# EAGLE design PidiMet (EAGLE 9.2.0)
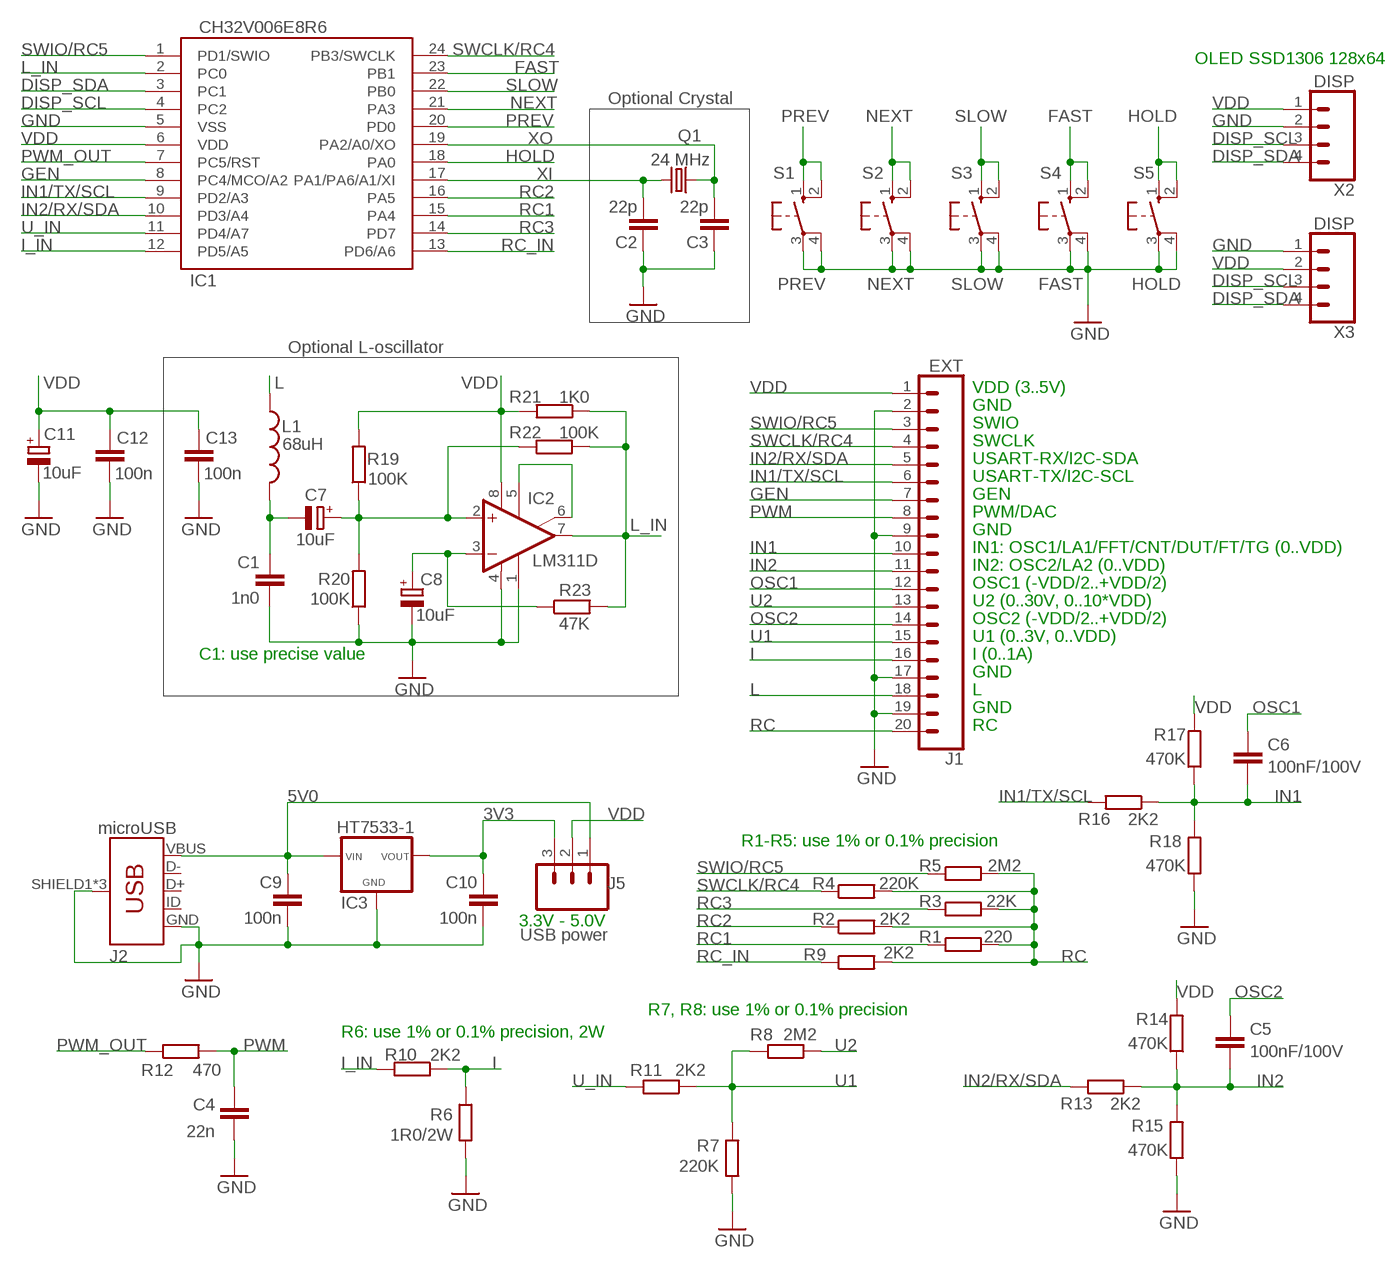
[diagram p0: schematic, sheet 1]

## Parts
C1  1n0  C5/2.5  [C5B2.5]
C2  22p  C-EUC1206  [C1206]
C3  22p  C-EUC1206  [C1206]
C4  22n  C-EUC1206  [C1206]
C5  100nF/100V  C-EUC1206  [C1206]
C6  100nF/100V  C-EUC1206  [C1206]
C7  10uF  CPOL-EUTT2D4L  [TT2D4L]
C8  10uF  CPOL-EUTT2D4L  [TT2D4L]
C9  100n  C-EUC1206  [C1206]
C10  100n  C-EUC1206  [C1206]
C11  10uF  CPOL-EUTT2D4L  [TT2D4L]
C12  100n  C-EUC1206  [C1206]
C13  100n  C-EUC1206  [C1206]
IC1  CH32V006E8R6  CH32V006E8R6CH32V006E8R6_2  [QSOP24_2]
IC2  LM311D  [SO08]
IC3  HT7533-1  [HT7533-1]
J1  EXT  CONN_201X20_LONGPADS  [1X20_LONGPADS]
J2  microUSB  USB_MICRO-B  [USB-B-MICRO-SMD_2]
J5  USB power  CONN_03LONGPADS  [1X03_LONGPADS]
L1  68uH  L-USLAL04  [LAL04]
Q1  24 MHz  CRYSTALHC49U-V  [HC49U-V]
R1  220  R-EU_0204/5  [0204/5]
R2  2K2  R-EU_0204/5  [0204/5]
R3  22K  R-EU_0204/5  [0204/5]
R4  220K  R-EU_0204/5  [0204/5]
R5  2M2  R-EU_0204/5  [0204/5]
R6  1R0/2W  R-EU_0414/15  [0414/15]
R7  220K  R-EU_0204/7  [0204/7]
R8  2M2  R-EU_0204/7  [0204/7]
R9  2K2  R-EU_R1206  [R1206]
R10  2K2  R-EU_R1206  [R1206]
R11  2K2  R-EU_R1206  [R1206]
R12  470  R-EU_R1206  [R1206]
R13  2K2  R-EU_R1206  [R1206]
R14  470K  R-EU_R1206  [R1206]
R15  470K  R-EU_R1206  [R1206]
R16  2K2  R-EU_R1206  [R1206]
R17  470K  R-EU_R1206  [R1206]
R18  470K  R-EU_R1206  [R1206]
R19  100K  R-EU_R1206  [R1206]
R20  100K  R-EU_R1206  [R1206]
R21  1K0  R-EU_R1206  [R1206]
R22  100K  R-EU_R1206  [R1206]
R23  47K  R-EU_R1206  [R1206]
S1  PREV  10-XX  [B3F-10XX]
S2  NEXT  10-XX  [B3F-10XX]
S3  SLOW  10-XX  [B3F-10XX]
S4  FAST  10-XX  [B3F-10XX]
S5  HOLD  10-XX  [B3F-10XX]
X2  DISP  CONN_04  [1X04]
X3  DISP  CONN_04  [1X04]

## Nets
3V3: C10.2 IC3.VOUT J5.3
5V0: C9.2 IC3.VIN J2.VBUS J5.1
DISP_SCL: IC1.4(PC2) X2.3 X3.3
DISP_SDA: IC1.3(PC1) X2.4 X3.4
FAST: IC1.23(PB1) S4.1(S) S4.2(S1)
GEN: IC1.8(PC4/MCO/A2) J1.7
GND: C1.2 C2.1 C3.1 C4.1 C8.- C9.1 C10.1 C11.- C12.1 C13.1 IC1.5(VSS) IC2.1(GND) IC2.4(V-) IC3.GND J1.2 J1.9 J1.17 J1.19 J2.GND J2.SHIELD1(SHIELD) J2.SHIELD2(SHIELD) J2.SHIELD3(SHIELD) R6.2 R7.2 R15.1 R18.1 R20.1 S1.3(P) S1.4(P1) S2.3(P) S2.4(P1) S3.3(P) S3.4(P1) S4.3(P) S4.4(P1) S5.3(P) S5.4(P1) X2.2 X3.1
HOLD: IC1.18(PA0) S5.1(S) S5.2(S1)
I: J1.16 R6.1 R10.1
I_IN: IC1.12(PD5/A5) R10.2
IN1: C6.2 J1.10 R16.1 R17.1 R18.2
IN1/TX/SCL: IC1.9(PD2/A3) J1.6 R16.2
IN2: C5.2 J1.11 R13.1 R14.1 R15.2
IN2/RX/SDA: IC1.10(PD3/A4) J1.5 R13.2
L: J1.18 L1.1
L_IN: IC1.2(PC0) IC2.7(OUT) R21.1 R22.2 R23.2
N$8: C7.+ IC2.2(+IN) R19.1 R20.2 R22.1
N$9: C1.1 C7.- L1.2
N$11: C8.+ IC2.3(-IN) R23.1
N$15: IC2.5(ON) IC2.6(ON/STR)
NEXT: IC1.21(PA3) S2.1(S) S2.2(S1)
OSC1: C6.1 J1.12
OSC2: C5.1 J1.14
PREV: IC1.20(PD0) S1.1(S) S1.2(S1)
PWM: C4.2 J1.8 R12.2
PWM_OUT: IC1.7(PC5/RST) R12.1
RC: J1.20 R1.2 R2.2 R3.2 R4.2 R5.2 R9.2
RC1: IC1.15(PA4) R1.1
RC2: IC1.16(PA5) R2.1
RC3: IC1.14(PD7) R3.1
RC_IN: IC1.13(PD6/A6) R9.1
SLOW: IC1.22(PB0) S3.1(S) S3.2(S1)
SWCLK/RC4: IC1.24(PB3/SWCLK) J1.4 R4.1
SWIO/RC5: IC1.1(PD1/SWIO) J1.3 R5.1
U1: J1.15 R7.1 R8.2 R11.1
U2: J1.13 R8.1
U_IN: IC1.11(PD4/A7) R11.2
VDD: C11.+ C12.2 C13.2 IC1.6(VDD) IC2.8(V+) J1.1 J5.2 R14.2 R17.2 R19.2 R21.2 X2.1 X3.2
XI: C2.2 IC1.17(PA1/PA6/A1/XI) Q1.2
XO: C3.2 IC1.19(PA2/A0/XO) Q1.1
Unconnected: J2.D+ J2.D- J2.ID

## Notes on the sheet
- OLED SSD1306 128x64
- Optional Crystal
- Optional L-oscillator
- VDD (3..5V)
- GND
- SWIO
- SWCLK
- USART-RX/I2C-SDA
- USART-TX/I2C-SCL
- GEN
- PWM/DAC
- GND
- IN1: OSC1/LA1/FFT/CNT/DUT/FT/TG (0..VDD)
- IN2: OSC2/LA2 (0..VDD)
- OSC1 (-VDD/2..+VDD/2)
- U2 (0..30V, 0..10*VDD)
- OSC2 (-VDD/2..+VDD/2)
- U1 (0..3V, 0..VDD)
- C1: use precise value | I (0..1A)
- GND
- L
- GND
- RC
- R1-R5: use 1% or 0.1% precision
- 3.3V - 5.0V
- R7, R8: use 1% or 0.1% precision
- R6: use 1% or 0.1% precision, 2W

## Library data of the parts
C1 = capacitor-wima:C: CAPACITOR
C2-C6 C9 C10 C12 C13 = rcl:C-EU: CAPACITOR, European symbol; SPICEPREFIX: C
C7 C8 C11 = rcl:CPOL-EU: POLARIZED CAPACITOR, European symbol; SPICEPREFIX: C
IC1 = CH32V:CH32V006E8R6
IC2 = linear:LM311: COMPARATOR
IC3 = HT7533-1B:HT7533-1
J1 = SparkFun-Connectors:CONN_20: Multi connection point. Often used as Generic Header-pin footprint for 0.1 inch spaced/style header connections On any of the 0.1 inch spaced packages, you can populate with these: Break Away Headers - Straight (PRT-00116) Break Away Male Headers - Right Angle (PRT-00553) Female Headers (PRT-00115)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
J2 = SparkFun-Connectors:USB_MICRO-B: USB Type Micro-B Connector Male/female and PTH/SMT variants SparkFun Products: SparkFun microB USB Breakout SparkFun USB microB Plug Breakout SparkFun ESP8266 Thing
J5 = SparkFun-Connectors:CONN_03: Multi connection point. Often used as Generic Header-pin footprint for 0.1 inch spaced/style header connections On any of the 0.1 inch spaced packages, you can populate with these: Break Away Headers - Straight (PRT-00116) Break Away Male Headers - Right Angle (PRT-00553) Female Headers (PRT-00115)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
L1 = rcl:L-US: INDUCTOR, American symbol; SPICEPREFIX: L
Q1 = crystal:CRYSTAL: CRYSTAL; OC_FARNELL: 1666969; OC_NEWARK: unknown
R1-R23 = rcl:R-EU_: RESISTOR, European symbol; SPICEPREFIX: R
S1-S5 = switch-omron:10-XX: OMRON SWITCH; MPN: B3F-1000; OC_FARNELL: 176432; OC_NEWARK: 36M3542
X2 X3 = SparkFun-Connectors:CONN_04: Multi connection point. Often used as Generic Header-pin footprint for 0.1 inch spaced/style header connections On any of the 0.1 inch spaced packages, you can populate with these: Break Away Headers - Straight (PRT-00116) Break Away Male Headers - Right Angle (PRT-00553) Female Headers (PRT-00115)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; PROD_ID: CONN-09696

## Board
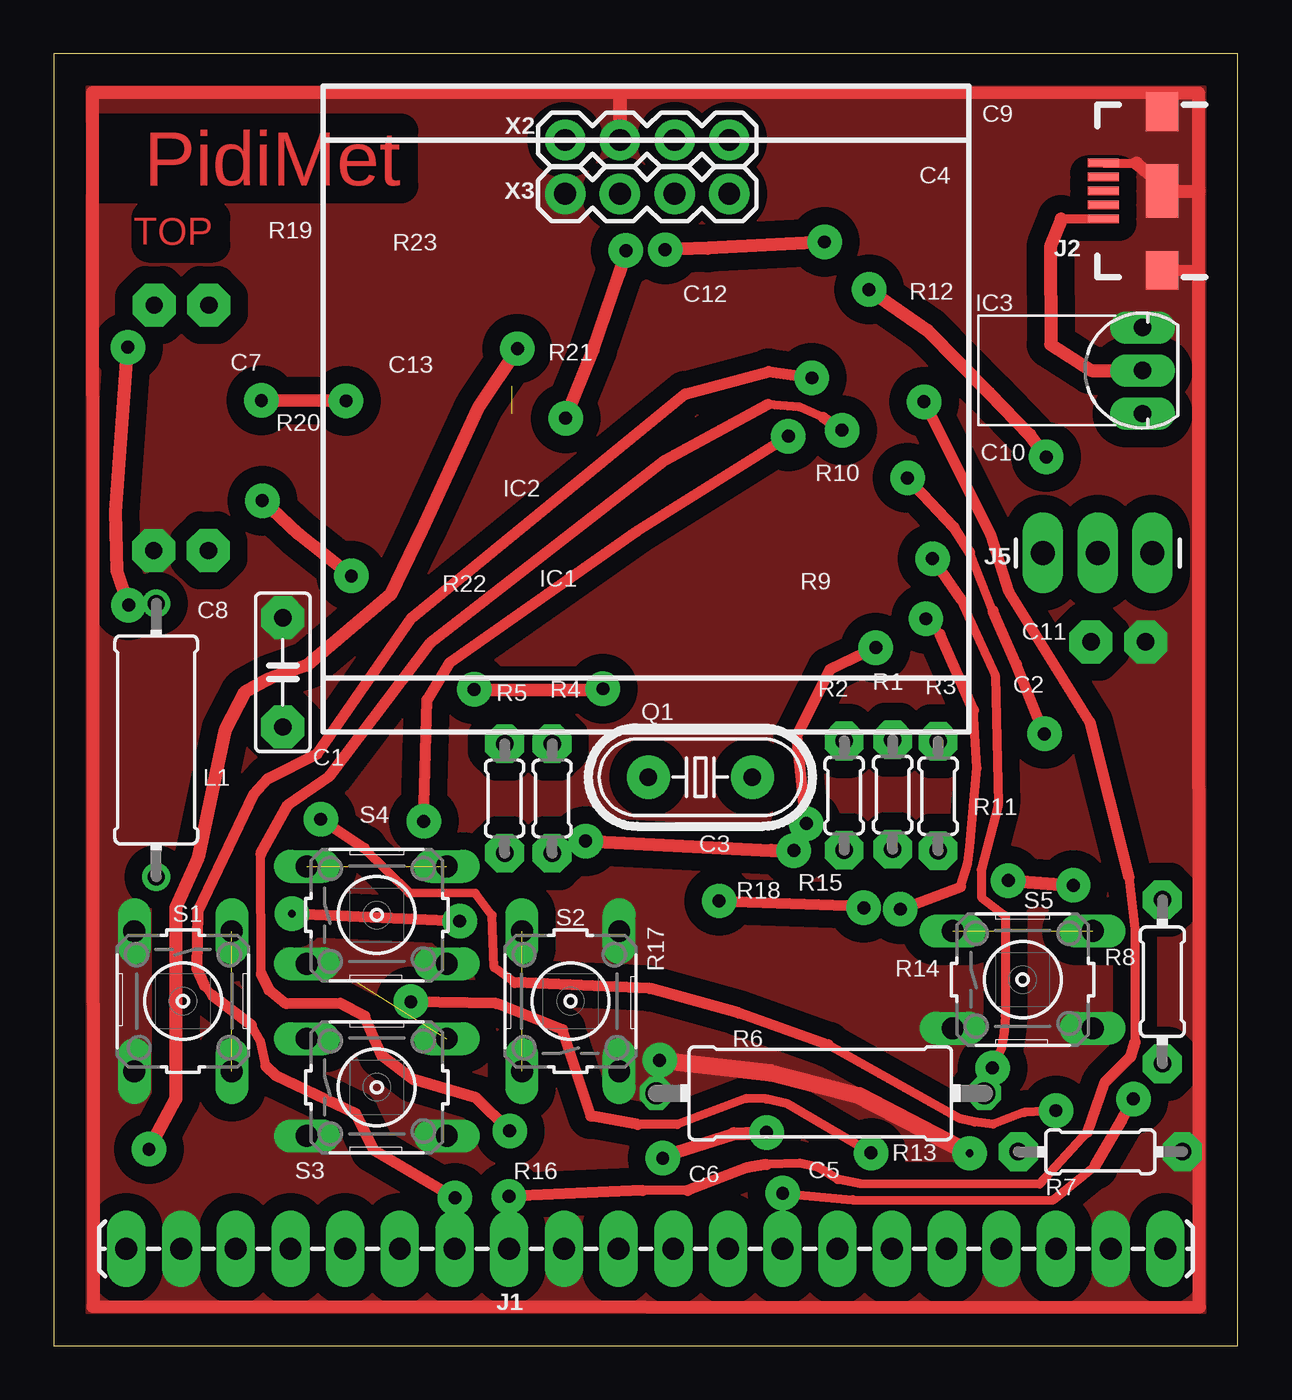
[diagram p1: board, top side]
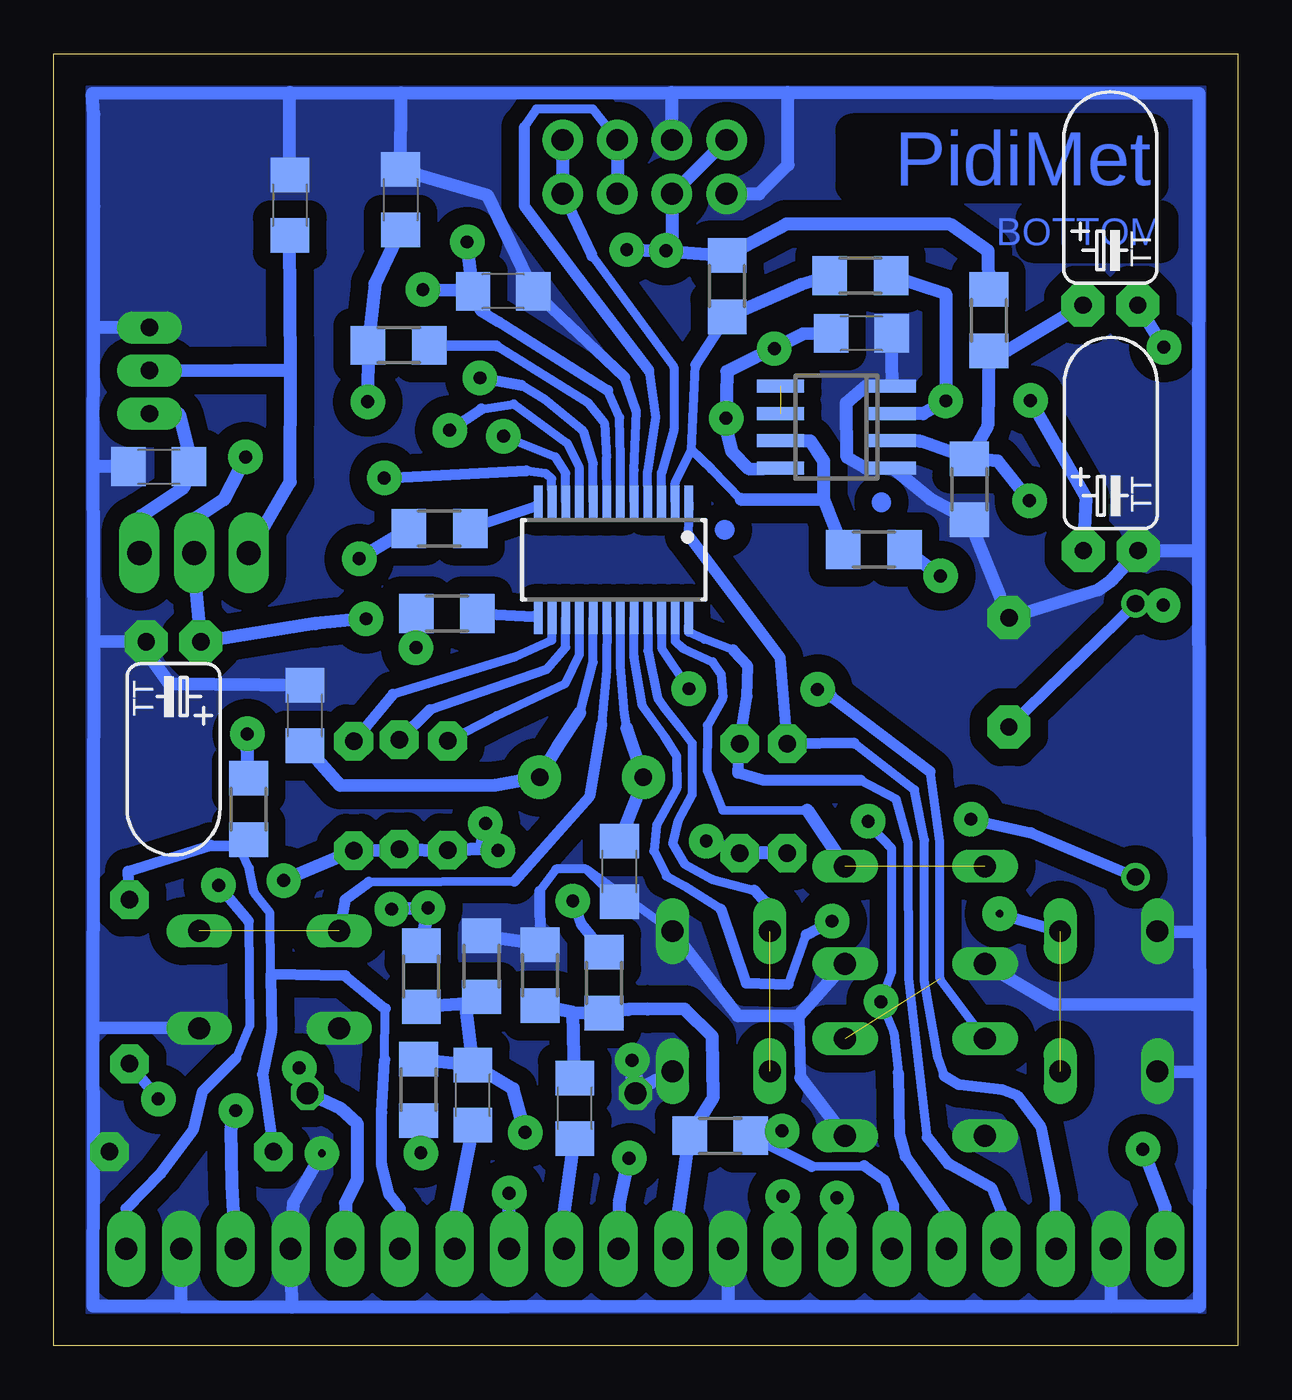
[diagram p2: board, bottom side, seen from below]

Size 55 x 60 mm. Coordinates in mm from the lower left corner, seen from the top.
Outline: 0,0 55,0 55,60 0,60 0,0
Copper layers (1*16): Top 0.035mm / dielectric 1.5mm / Bottom 0.035mm
Design rules "default": minimum track width 6mil, minimum drill 0.35mm, track to track 6mil, track to pad 6mil, pad to pad 6mil, via to via 6mil, smd to smd 6mil, copper to edge 40mil, drill to drill 6mil, minimum pad ring 10mil, minimum via ring 8mil, stop-mask expansion 4mil, vias tented up to drill 0mil, thermal gap 10mil

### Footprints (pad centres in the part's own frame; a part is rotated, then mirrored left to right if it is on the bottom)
C5B2.5 = drill 0.8 pad 2 octagon: 1 -2.54,0 | drill 0.813 pad 2 octagon: 2 2.54,0
C1206 = smd 1.6 x 1.8: 1 -1.4,0; 2 1.4,0
TT2D4L = drill 0.8 pad 2 octagon: + -1.27,0; - 1.27,0
QSOP24_2 = smd 0.4 x 1.5: 1 -3.493,-2.69; 2 -2.857,-2.69; 3 -2.223,-2.69; 4 -1.587,-2.69; 5 -0.953,-2.69; 6 -0.318,-2.69; 7 0.318,-2.69; 8 0.953,-2.69; 9 1.587,-2.69; 10 2.223,-2.69; 11 2.857,-2.69; 12 3.493,-2.69; 13 3.493,2.69; 14 2.857,2.69; 15 2.223,2.69; 16 1.587,2.69; 17 0.953,2.69; 18 0.318,2.69; 19 -0.318,2.69; 20 -0.953,2.69; 21 -1.587,2.69; 22 -2.223,2.69; 23 -2.857,2.69; 24 -3.493,2.69
SO08 = smd 0.6 x 2.2: 1 -1.905,-2.6; 2 -0.635,-2.6; 3 0.635,-2.6; 4 1.905,-2.6; 5 1.905,2.6; 6 0.635,2.6; 7 -0.635,2.6; 8 -1.905,2.6
HT7533-1 = drill 0.8 pad 1.5 long: GND 2,0; VIN 0,0; VOUT -2,0
1X20_LONGPADS = drill 1.016 pad 1.778 long: 1 -24.13,0; 2 -21.59,0; 3 -19.05,0; 4 -16.51,0; 5 -13.97,0; 6 -11.43,0; 7 -8.89,0; 8 -6.35,0; 9 -3.81,0; 10 -1.27,0; 11 1.27,0; 12 3.81,0; 13 6.35,0; 14 8.89,0; 15 11.43,0; 16 13.97,0; 17 16.51,0; 18 19.05,0; 19 21.59,0; 20 24.13,0
USB-B-MICRO-SMD_2 = smd 1.45 x 0.4: D+ 2.725,0; D- 2.725,0.65; GND 2.725,-1.3; ID 2.725,-0.65; VBUS 2.725,1.3 | smd 1.5 x 1.8: SHIELD1 0,3.685; SHIELD2 0,-3.685 | smd 1.5 x 2.5: SHIELD3 0,0
1X03_LONGPADS = drill 1.118 pad 1.88 long: 1 0,0; 2 2.54,0; 3 5.08,0
LAL04 = drill 0.8 pad 1.3: 1 -6.35,0; 2 6.35,0
HC49U-V = drill 0.813 pad 2: 1 -2.413,0; 2 2.413,0
0204/5 = drill 0.813 pad 1.8 octagon: 1 -2.54,0; 2 2.54,0
0414/15 = drill 1.016 octagon: 1 -7.62,0; 2 7.62,0
0204/7 = drill 0.813 pad 1.8 octagon: 1 -3.81,0; 2 3.81,0
R1206 = smd 1.6 x 1.803: 1 -1.422,0; 2 1.422,0
B3F-10XX = drill 1.016 long: 1 -3.251,2.261; 2 3.251,2.261; 3 -3.251,-2.261; 4 3.251,-2.261
1X04 = drill 1.016 pad 1.88: 1 0,0; 2 2.54,0; 3 5.08,0; 4 7.62,0

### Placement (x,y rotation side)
C1  10.64,31.27 90 top
C2  43.34,29.27 270 bottom
C3  28.73,22.03 90 bottom
C4  38.89,53.23 270 bottom
C5  35.54,11.64 90 bottom
C6  30.8,11.02 90 bottom
C7  5.93,48.33 0 bottom
C8  5.91,36.93 0 bottom
C9  44.04,52.97 270 bottom
C10  50.13,40.82 0 bottom
C11  49.44,32.69 180 bottom
C12  34.13,48.97 180 bottom
C13  17.49,47.01 180 bottom
IC1  29,36.5 180 bottom
IC2  18.65,42.66 90 bottom
IC3  50.56,45.29 90 top
J1  27.5,4.5 0 top
J2  51.47,53.63 180 top
J5  45.94,36.82 0 top
L1  4.76,28.12 90 top
Q1  30.03,26.4 0 top
R1  38.96,25.6 270 top
R2  36.71,25.55 270 top
R3  41.07,25.53 270 top
R4  23.14,25.41 270 top
R5  20.94,25.42 270 top
R6  35.6,11.72 180 top
R7  48.61,9.01 0 top
R8  51.49,16.9 90 top
R9  36.75,34.01 180 bottom
R10  37.08,37.95 0 bottom
R11  45.95,24.93 90 bottom
R12  38.99,46.46 180 bottom
R13  38.06,11.88 270 bottom
R14  37.93,17.16 90 bottom
R15  35.13,17.62 270 bottom
R16  24.05,9.75 0 bottom
R17  29.44,16.86 90 bottom
R18  32.42,17.21 270 bottom
R19  11.57,47.63 90 bottom
R20  12.48,39.77 90 bottom
R21  23.72,49.21 90 bottom
R22  16.91,36.98 180 bottom
R23  17.54,49.7 180 bottom
S1  6,16 270 top
S2  24,16 90 top
S3  15,12 0 top
S4  15,20 0 top
S5  45,17 0 top
X2  23.75,56 0 top
X3  23.75,53.5 0 top

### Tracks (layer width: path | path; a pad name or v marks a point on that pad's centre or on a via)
3V3
  Bottom 0.61: J5.3 50.92,38.56 48.95,39.89 C10.2 48.78,41.68 49.19,43.27 IC3.VOUT
5V0
  Top 0.406: J2.VBUS 46.79,52.33
  Top 0.61: 46.79,52.33 46.29,51.06 46.3,46.5 48.19,45.29 IC3.VIN
  Bottom 0.61: IC3.VIN 46.59,45.3 44.01,45.3 | J5.1 44.02,40.13 44.01,45.3 | 44.01,45.3 C9.2
DISP_SCL
  Bottom 0.406: IC1.4 27.42,40.63 27.05,43.13 27.36,45.29 | X2.3 29.97,57.43 32.58,57.43 33.15,56.59
  Bottom 0.508: 33.15,56.59 33.15,52.94 30.95,50 27.36,45.29
  Bottom 0.61: X2.3 X3.3
DISP_SDA
  Bottom 0.406: IC1.3 26.78,40.53 26.2,42.54 26.2,45.45 30.01,50.62
  Bottom 0.508: X3.4 30.01,50.62
  Bottom 0.61: X2.4 X3.4
FAST  (1 unrouted)
  Bottom 0.406: IC1.23 26.14,32.72 25.77,32.38 24.4,31.76 24.01,31.19 23.93,30.09 24.65,28.81 24.65,26.7 23.93,24.87 20,24.87
  Bottom 0.61: 20,24.87 S4.2
GEN  (via drill 0.6 pad 1.6)
  Top 0.406: 9.86,12.98 9.61,14.14 9.18,14.9 | 7.36,16.27 7,16.73
  Top 0.508: v18.63,6.86 14.85,9.1 14.03,10.77 10.32,12.53 9.86,12.98 | 9.18,14.9 7.36,16.27 | 7,16.73 6.66,17.5 6.7,20.18 9.28,25.6 9.96,26.35 12.24,27.5 16.63,33.81 29.32,44.2 33.21,45.25 v35.2,44.95
  Bottom 0.406: IC1.8 29.95,40.97 30.43,42.49 32.2,43.96 33.28,44.61
  Bottom 0.508: J1.7 v18.63,6.86 | v35.2,44.95 33.28,44.61
GND  (via drill 0.35 pad 1.6, 0.6 pad 1.6)
  Top 0.406: J2.GND 50.29,54.93
  Top 0.508: J2.SHIELD2 51.45,58.17 | J2.SHIELD3 51.85,53.62 | J2.SHIELD1 53.18,49.94
  Top 0.61: 53.19,53.62 53.18,49.94 53.21,1.79 1.82,1.82 1.79,58.2 26.3,58.2 X2.2 26.29,57.99 | 53.19,53.62 53.17,58.17 51.45,58.17 26.3,58.19 26.34,58.03 | 53.19,53.62 51.85,53.62 50.29,54.93
  Top 0.813: v42.54,8.93 37.42,11.61 33.28,12.67 v28.14,13.25
  Bottom 0.406: C11.- 51.02,32.68 | IC1.5 28.04,40.67 27.94,43.39 28.48,44.98 | S2.4 30.29,22.14 | 30.29,22.14 31.68,22.14 32.43,21.11 | C3.1 30.29,22.14 | 2.1,15.85 1.78,15.81
  Bottom 0.508: 28.48,44.98 C12.1 | 32.43,21.11 R18.1 | 20.38,15.34 20.32,12.46
  Bottom 0.61: J1.19 49.11,1.83 | 49.11,1.83 43.95,1.8 | 43.95,1.8 23.7,1.86 | 23.7,1.86 5.88,1.83 | 5.88,1.83 J1.2 | J1.9 23.7,1.86 | 43.95,1.8 J1.17 43.86,6.62 v42.54,8.93 | 49.11,1.83 53.18,1.83 53.16,8.99 | 53.16,8.99 53.16,14.75 | 53.16,14.75 53.14,32.71 | 53.14,32.71 53.18,40.84 | 53.18,40.84 53.15,47.28 | 53.15,47.28 53.15,49.9 53.14,52.9 53.14,57.18 53.21,58.16 44.04,58.2 | 44.04,58.2 38.88,58.17 | 38.88,58.17 26.3,58.2 | 26.3,58.2 20.91,58.21 | 20.91,58.21 1.82,58.16 1.83,36.94 | 1.83,36.94 1.79,19.22 | 1.79,19.22 1.78,15.81 1.77,12.72 | 1.77,12.72 1.79,1.82 5.88,1.83 | S1.3 1.79,19.22 | S1.4 1.77,12.72 | S5.4 53.16,14.75 | IC3.GND 53.15,47.28 | C10.1 53.18,40.84 | 53.14,32.71 51.02,32.68 49.62,30.72 C2.1 | X2.2 26.3,58.2 | X3.1 22.24,53.5 20.89,54.85 20.91,58.21 | 27.95,11.84 S2.3 | R18.1 R15.1 | R7.2 53.16,8.99 | 1.83,36.94 C8.- 5.86,35.57 6.48,35.11 C1.2 R20.1 14.28,39.32 IC2.1 17.31,40.77 18.16,41.25 18.2,43.8 17.23,44.6 IC2.4 C13.1 | C12.1 34.86,53.43 C4.1 38.88,58.17 | S4.4 20.38,15.34 23.23,15.32 S2.4 | 20.32,12.46 S3.4 | S4.3 8.59,15.88 2.1,15.85 | C9.1 44.04,58.2
  Bottom 0.813: R6.2 27.95,11.84 v28.14,13.25
  pour Bottom (isolate 0.813, no thermals): 1.5,1.5 1.5,58.5 53.5,58.5 53.5,1.5
  pour Top (isolate 0.813, no thermals): 1.5,58.5 53.5,58.5 53.5,1.5 1.5,1.5
HOLD  (1 unrouted)
  Bottom 0.406: IC1.18 29.32,31.38 29.56,28.86 | 33.62,21.57 40.36,21.52
  Bottom 0.508: 29.56,28.86 30.13,25.5 33.62,21.57 | 40.36,21.52 41.48,20.7 S5.1
I  (via drill 0.6 pad 1.6)
  Top 0.406: 42.12,34.69 43.73,31.13 43.87,25.14 43.08,22.12 43.09,20.82 44.19,19.97 44.18,15.32 44.14,14.63 44.02,13.81 v43.6,12.89
  Top 0.508: v40.81,36.55 42.12,34.69
  Bottom 0.61: J1.16 41.45,6.63 40.9,7.74 40.89,10.29 41.65,10.99 R6.1 | R10.1 v40.81,36.55
  Bottom 0.813: R6.1 v43.6,12.89
I_IN
  Bottom 0.406: IC1.12 32.67,38.96
  Bottom 0.508: 32.67,38.96 R10.2
IN1
  Bottom 0.61: C6.2 30.87,15.47 | 30.87,15.47 R18.2 | 30.87,15.47 R17.1 28.32,15.61 27.42,15.64 25.69,15.63 24.41,14.36 24.36,11.54 R16.1 J1.10
IN1/TX/SCL  (via drill 0.6 pad 1.6)
  Top 0.406: 9.63,17.28 9.62,22.83 | 33.17,43.73 34.63,43.61 35.73,43.12
  Top 0.508: v21.17,9.97 19.6,11.52 16.69,12.37 15.22,13.48 14.45,15.3 13.3,15.9 10.79,15.88 9.99,16.51 9.63,17.28 | 9.62,22.83 10.89,25.13 12.8,26.47 17.51,32.65 28.38,41.13 33.17,43.73 | 35.73,43.12 v36.61,42.52
  Bottom 0.406: 19.79,8.33 17.36,8.36 | IC1.9 30.59,40.75 31.15,41.91 33.63,43.73 35.13,43.51 | R16.2 v21.17,9.97
  Bottom 0.508: R16.2 19.79,8.33 | 17.36,8.36 16.43,7.7 16,6.53 J1.6 | v36.61,42.52 35.13,43.51
IN2  (via drill 0.6 pad 1.6)
  Top 0.406: v28.28,8.71 28.44,8.84
  Top 0.61: 28.44,8.84 31.58,9.84 v33.11,9.9
  Bottom 0.406: 35.88,15.87 R15.2
  Bottom 0.61: C5.2 35.88,15.87 R14.1 | J1.11 28.71,6.66 v28.28,8.71 | v33.11,9.9 33.66,11.93 C5.2 | R13.1 C5.2
IN2/RX/SDA  (via drill 0.6 pad 1.6)
  Top 0.406: v37.95,8.95 34.07,11.23 33.08,11.46 32.16,11.48 28.97,10.27 27.12,10.27
  Top 0.508: 27.12,10.27 24.95,10.67 23.64,14.68 20.56,15.89 v16.58,15.97 | v17.18,24.35 17.33,29.99 18.38,31.73 27.04,37.81 v34.12,42.24
  Bottom 0.406: 15.78,12.67 15.99,14.54 v16.58,15.97 16.08,17.35 16.08,23.08 16.94,24.01 v17.18,24.35 | IC1.10 31.22,40.53 31.71,41.28 v34.12,42.24
  Bottom 0.508: R13.2 v37.95,8.95 | 15.78,12.67 15.72,9.78 15.46,8.78 13.49,6.05 J1.5
L  (via drill 0.6 pad 1.6)
  Top 0.406: v46.55,10.92 45.06,10.83 43.62,10.28 42.76,10.39 42.09,10.54 35.96,13.98 | 21.41,16.87 20.46,17.56 20.36,19.99 19.58,21.01 16.52,21.02 14.42,23.09
  Top 0.508: 35.96,13.98 31.8,15.45 27.68,16.59 21.41,16.87 | 14.42,23.09 v12.4,24.45
  Bottom 0.508: v12.4,24.45 9.6,23.82 L1.1
  Bottom 0.61: J1.18 46.72,7.48 46.76,10.1 v46.55,10.92
L_IN
  Bottom 0.406: IC1.2 26.15,40.07 25.37,41.6 | 23.08,39.3 24.46,40.71 25.37,41.6 | 25.37,41.6 25.2,45.55
  Bottom 0.508: 25.2,45.55 R21.1
  Bottom 0.61: IC2.7 19.87,42.03 19.25,41.09 19.26,39.31 | 19.26,39.31 R22.2 | R21.1 20.28,49.3 R23.2 | 23.08,39.3 19.26,39.31
N$8  (via drill 0.6 pad 1.6)
  Top 0.406: 9.72,39.25 v9.68,39.25
  Top 0.61: v13.82,35.75 11.37,37.7 9.72,39.25
  Bottom 0.61: C7.+ 10.71,46.22 R19.1 11.62,42.74 R20.2 | R20.2 14.76,42 IC2.2 | R22.1 v13.82,35.75 | v9.68,39.25 11.16,41.1 R20.2
N$9  (via drill 0.6 pad 1.6)
  Top 0.61: v3.48,34.4 2.94,35.98 2.87,38.74 v3.44,46.37
  Bottom 0.508: L1.2 C1.1
  Bottom 0.61: L1.2 v3.48,34.4 | v3.44,46.37 C7.-
N$11  (via drill 0.6 pad 1.6)
  Top 0.406: 9.65,43.86 v9.64,43.9
  Top 0.61: v13.57,43.88 9.65,43.86
  Bottom 0.61: R23.1 13.57,48.85 v13.57,43.88 14.62,43.28 IC2.3 | v9.64,43.9 7.07,39.4 C8.+
N$15  (1 unrouted)
NEXT  (1 unrouted)
  Bottom 0.406: IC1.21 27.41,32.27 26.95,30.09 26.57,29.52 25.91,28.7 25.35,27.97 25.35,25.6 26,24.39 26.26,23.33 25.71,22.38 24.42,21.66 22.46,21.14
  Bottom 0.508: 22.46,21.14 22.11,20.75 21.73,20.48 S2.2
OSC1
  Bottom 0.61: J1.12 31.3,6.11 C6.1
OSC2
  Bottom 0.61: C5.1 36.36,6.02 J1.14
PREV  (via drill 0.35 pad 1.6, 0.6 pad 1.6)  (1 unrouted)
  Top 0.508: v18.85,19.72 v11.06,20.06
  Bottom 0.406: IC1.20 28.05,31.99 27.66,29.69 26.62,28.25 26.07,27.38 26.06,25.89 27,24.19 27.12,22.97 26.55,21.81 25.7,21.35 24.02,20.28 | 20.88,16.78 20.06,19.08
  Bottom 0.508: v11.06,20.06 S1.1 | 24.02,20.28 22.84,16.84 20.88,16.78 | 20.06,19.08 v18.85,19.72
PWM  (via drill 0.6 pad 1.6)
  Top 0.406: 49.93,21.75 50.21,19.36 50.22,14.11 | 48.01,9.92 45.78,7.5 37.46,7.52 36.41,7.72 35.52,8.28 34.65,8.48 33.11,8.42 | 29.45,7.21 27.35,7.21
  Top 0.508: v40.42,43.84 43.52,37.64 44.37,35 48.13,28.95 49.93,21.75 | 50.22,14.11 50.01,13.41 48.8,12.2 48.01,9.92 | 33.11,8.42 32.18,8.26 29.45,7.21 | 27.35,7.21 v21.14,6.93
  Bottom 0.508: v21.14,6.93 J1.8
  Bottom 0.61: C4.2 40.08,49.33 R12.2 v40.42,43.84
PWM_OUT
  Bottom 0.406: IC1.7 29.33,41.21 29.42,42.85 30.19,43.8 34.45,46.44
  Bottom 0.508: R12.1 34.45,46.44
RC  (via drill 0.6 pad 1.6)
  Top 0.508: v38.18,32.42 36.04,31.4 34.48,28.32 34.87,24.69
  Top 0.61: v24.7,23.44 33.31,23.01 v34.37,23 | v44.33,21.6 v47.35,21.38 | 34.87,24.69 v34.95,24.25
  Bottom 0.406: 24.57,23.44 v24.7,23.44 | 45.95,19.73 45.89,14.87 46.53,13.36
  Bottom 0.508: v47.35,21.38 45.95,19.73 | 46.53,13.36 48.1,11.79 48.52,10.03 50.04,7.99 51.64,6.37 J1.20
  Bottom 0.61: R5.2 R4.2 24.57,23.44 | v34.37,23 35.15,23.08 | 35.15,23.08 R2.2 R1.2 R3.2 v44.33,21.6 | R9.2 v38.18,32.42 | v34.95,24.25 35.15,23.08
RC1
  Bottom 0.406: 37.53,29.55 32.1,31.42 31.22,32.44 IC1.15
  Bottom 0.508: R1.1 37.53,29.55
RC2
  Bottom 0.406: R2.1 34.45,29.25 31.24,30.76 30.59,32.09 IC1.16
RC3
  Bottom 0.406: 39.24,30.26 33.55,32.01 31.86,32.77 IC1.14
  Bottom 0.508: R3.1 39.24,30.26
RC_IN
  Bottom 0.406: 32.7,33.87 IC1.13
  Bottom 0.508: R9.1 32.7,33.87
SLOW  (via drill 0.6 pad 1.6)  (1 unrouted)
  Top 0.61: v19.53,30.48 24.86,30.45 v25.5,30.51
  Bottom 0.406: IC1.22 26.77,32.41 v25.5,30.51 | S3.1 13.84,17.04 13.85,23.42 14.29,26.66
  Bottom 0.508: 14.29,26.66 18.89,30.13
  Bottom 0.61: 18.89,30.13 v19.53,30.48
SWCLK/RC4
  Bottom 0.406: 23.45,32.31 24.8,32.82 25.52,33.14 IC1.24 | 14.43,9.66 15.29,17.07 15.31,23.34 15.87,25.37 17.54,26.26
  Bottom 0.508: 23.45,32.31 22.77,31.56 22.8,30.15 R4.1 23.23,26.59 22.05,26.26 17.54,26.26 | J1.4 11.01,6.29 11.41,7.3 13.46,8.44 14.43,9.66
SWIO/RC5
  Bottom 0.406: IC1.1 25.55,37.65 | 13.65,12.54 13.95,13.37 14.57,16.93 14.56,23.47 15.02,25.82 17.84,27.98
  Bottom 0.508: 25.55,37.65 21.26,31.94 R5.1 17.84,27.98 | J1.3 8.49,6.9 9.13,10.13 10.23,11.59 10.96,11.88 12.94,12.12 13.65,12.54
U1
  Bottom 0.406: 39.63,13.28 39.61,15.65 | 44.92,17.24 44.96,20.09 45.7,21.04 45.92,22.18 46.42,23.2 R11.1
  Bottom 0.508: J1.15 38.9,6.36 39.43,7.02 39.77,8.41 39.77,10.83 39.63,13.28 | 39.61,15.65 41.47,17.18 44.92,17.24 44.89,14.62 45.3,12.59 R7.1 | R8.2 51.55,22.04 47.7,23.24 46.42,23.2
U2  (via drill 0.6 pad 1.6)
  Top 0.406: v33.85,7.08 37.1,6.78 46.39,6.76 48.36,8.32
  Top 0.508: 48.36,8.32 49.58,10.44 v50.15,11.46
  Bottom 0.508: v50.15,11.46 R8.1
  Bottom 0.61: J1.13 33.86,6.8 v33.85,7.08
U_IN  (via drill 0.6 pad 1.6)
  Top 0.406: 43.62,34.13 42.54,36.84
  Top 0.508: v46.01,28.42 44.72,31.64 43.62,34.13 | 42.54,36.84 41.8,38 v39.65,40.3
  Bottom 0.406: IC1.11 31.87,40.27 32.16,40.52 33.05,40.64 | 46.05,28.42 v46.01,28.42
  Bottom 0.508: v39.65,40.3 33.05,40.64
  Bottom 0.61: R11.2 46.05,28.42
VDD  (via drill 0.6 pad 1.6)
  Top 0.406: 4.47,9.25 v4.42,9.13 | 36.88,20.44 v37.62,20.33 | 42.11,21.31 42.45,22.41 42.54,23.19 42.87,26.83 42.72,29.51 | 41.16,33.05 v40.5,33.76
  Top 0.508: v30.9,20.66 36.88,20.44 | v39.31,20.27 42.11,21.31 | 42.72,29.51 41.16,33.05
  Top 0.61: v23.77,43.08 25.05,46.25 26.24,49.76 v26.57,50.87 | v21.53,46.31 19.71,43.56 17.09,37.88 15.63,34.88 11.78,31.6 9.96,30.95 8.87,30.35 7.96,28.63 6.7,22.67 5.67,20.36 5.66,11.46 4.47,9.25 | v35.8,51.26 30.38,50.97 v28.39,50.91 | v37.86,49.06 40.6,47.15 43.45,44.25 45.33,42.3 v46.09,41.27
  Bottom 0.406: J5.2 48.54,36.68 | IC1.6 28.68,41.25 28.71,43.11 29.27,44.37 | 21.68,46.18 v21.53,46.31 | 35.8,51.18 v35.8,51.26
  Bottom 0.508: 29.27,44.37 34.33,47.55 35.19,48.07 C12.2 | R17.2 30.5,19.57 v30.9,20.66
  Bottom 0.61: X2.1 X3.2 26.3,51.35 26.49,50.84 | C13.2 20.22,46.99 v21.53,46.31 22.42,45.9 23.74,45.24 v23.77,43.08 23.76,42.51 23.52,41.55 22.7,40.72 IC2.8 | 26.49,50.84 R21.2 20.98,52.09 13.36,52.09 11.6,50.84 R19.2 | v26.57,50.87 26.76,50.86 | 26.76,50.86 26.49,50.84 | v4.42,9.13 3.39,6.42 J1.1 | 35.8,51.18 C12.2 v37.86,49.06 | v28.39,50.91 26.76,50.86 | v46.09,41.27 47.1,39.3 48.46,38.39 48.54,36.68 C11.+ 42.86,33.53 v40.5,33.76 | R14.2 v37.62,20.33 v39.31,20.27
XI
  Bottom 0.406: 30.57,29.39 29.95,31.73 IC1.17
  Bottom 0.61: 30.57,29.39 31.6,27.81 Q1.2 34.49,26.03 41.7,26.02 C2.2
XO
  Bottom 0.406: Q1.1 27.71,26.66 | 28.39,28.67 28.5,29.33 28.69,31.56 IC1.19
  Bottom 0.61: 28.39,28.67 27.71,26.66 27.72,25.95 C3.2
(copper drawn outside any net)
  shapes: Bottom circle x2

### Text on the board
Top: PidiMet | TOP
Bottom: PidiMet | BOTTOM
Document: VCC-GND | GND-VCC | 5V | 3V3 | GND | VDD | SWDIO | 1 | 5 | 10 | 15 | 20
